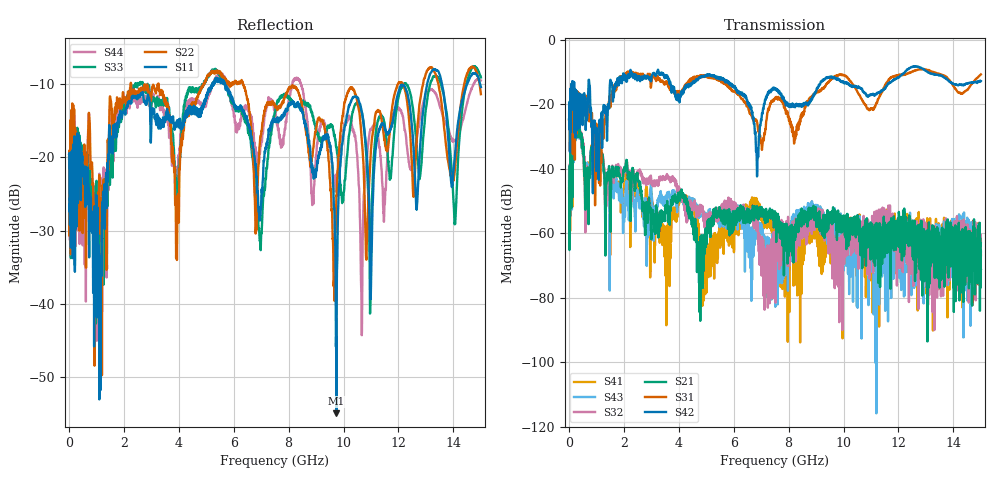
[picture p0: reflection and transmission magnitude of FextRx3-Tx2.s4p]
! FILE: N:\QM 2007\Prüfprotokolle\Highspeed\Konfektionierte Ltg\L45593-D106\D30\8216\0002\Fext\FextRx3-Tx2.s4p
# MHz S DB R 50.00
! FREQ  S11  S12  S13  S14
!  S21  S22  S23  S24
!  S31  S32  S33  S34
!  S41  S42  S43  S44
!  DB  ANG  DB  ANG  DB  ANG  DB  ANG
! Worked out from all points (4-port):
!   2999 points, 10 MHz to 15 GHz, reference 50 ohm
!   strongest paths, dB at 10 MHz, 3.755 GHz, 7.505 GHz, 11.26 GHz, 15 GHz:
!     S42: -24.6, -14.9, -15.1, -16.4, -12.8
!     S31: -24.7, -15.7, -18.1, -18.4, -10.7
!     S21: -43.9, -50.5, -54.5, -60.6, -71.1
!     S32: -47.3, -42.9, -65.2, -55.5, -62.8
!     S43: -41.5, -48.7, -62.6, -76.6, -65.7
!     S41: -46.1, -53.2, -60.1, -64.4, -66.8
!   lowest |S11| = -55.0 dB at 9.74 GHz (marker M1), VSWR 1.00, Z = 50 + j0.178 ohm
!   |S11| at or under -10 dB: start of sweep to 5.213 GHz; 5.693 GHz to 13.04 GHz (7.348 GHz wide, 78.4 % of centre); 13.58 GHz to 14.49 GHz (907.6 MHz wide, 6.46 % of centre)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
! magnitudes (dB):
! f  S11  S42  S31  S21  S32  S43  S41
! 10 MHz  -19.5  -24.6  -24.7  -43.9  -47.3  -41.5  -46.1
! 320 MHz  -19.8  -22.8  -19.6  -29.2  -28.5  -29.1  -29.1
! 4.81 GHz  -13.3  -11.3  -11.4  -70.6  -52.5  -53.0  -76.1
! 6.87 GHz  -24.7  -36.4  -26.4  -53.9  -56.4  -59.2  -51.3
! 9.74 GHz  -55.0  -12.3  -11.0  -56.8  -61.8  -57.9  -66.6
! 10.34 GHz  -11.8  -14.2  -13.7  -57.4  -59.9  -70.2  -63.8
! 15 GHz  -10.4  -12.8  -10.7  -71.1  -62.8  -65.7  -66.8
